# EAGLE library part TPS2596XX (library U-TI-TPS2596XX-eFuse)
TPS2596XX - eFuse With Accurate Current Monitor and Fast Overvoltage Protection Specifications Input voltage: 2.7-V to 19-V, (21-V Absolute maximum) Overvoltage Protection: Fast overvoltage clamp (3.8-V, 5.7-V and 13.8- V pin-selectable thresholds) with a response time of 5-μs (typical) Current Limiting: Adjustable, 0.125-A to 2-A Current Monitoring: Analog through pin ILIM Operating Temperature Range: –40 °C to +125 °C Body Size: SOIC (8) 4.91 mm x 3.9 mm
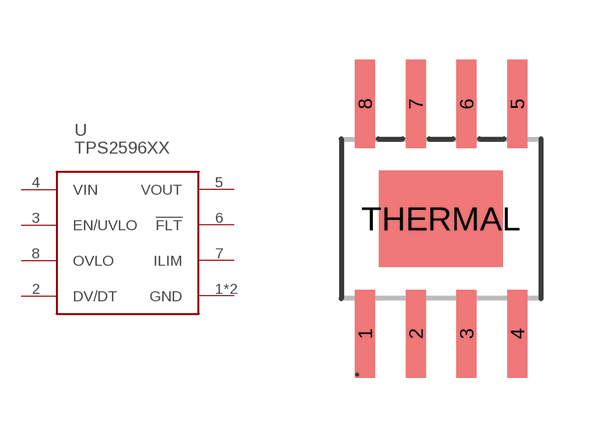
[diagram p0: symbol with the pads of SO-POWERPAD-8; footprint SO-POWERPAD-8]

Designator prefix -

## TPS2596XX  [SO-POWERPAD-8]
1  GND
2  DV/DT
3  EN/UVLO
4  VIN  pwr
5  VOUT  pwr
6  !FLT
7  ILIM
8  OVLO
THERMAL  GND

## Footprint SO-POWERPAD-8 (pad centres in mm)
smd 0.5 x 2.2: 1 -1.905,-2.875; 2 -0.635,-2.875; 3 0.635,-2.875; 4 1.905,-2.875; 5 1.905,2.875; 6 0.635,2.875; 7 -0.635,2.875; 8 -1.905,2.875
smd 3.1 x 2.4: THERMAL 0,0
